FUNCTION_BLOCK FB111
TITLE =Get Velocity Must
//*****************************************************************************
//* maxon motor ag
//* R&D
//* all rights reserved
//*****************************************************************************
//* Summary:  Read demand value of velocity
//*
//* Remarks:
//*
//* Created under: STEP7 REV5.2+SP1
//*****************************************************************************
//* History:
//* 19.05.2004 | INA   first release
//*
//*
//*****************************************************************************
//

AUTHOR:INA
FAMILY:Velocity
NAME:SetVeloM
VERSION:00.01


VAR_INPUT

Read : BOOL //A rising edge start the command

  NodeID : BYTE //Adress of the maxon device

END_VAR
VAR_OUTPUT
  Done : BOOL //Data valid flag is TRUE if data were available

  Err : BOOL //Error flag is TRUE if an Error has occured, see ErrNo for more details

  ErrNo : DINT //Contains detailed error information

  VelocityMust : DINT //Velocity demand value

END_VAR
VAR
  xEdgeMerker : BOOL //Edge Merker

  xEdgeFlag : BOOL //Edge Flag

  xStep : INT
END_VAR

BEGIN

NETWORK
TITLE = Activate the service function
//

// SDO Read "Get Velocity Must"

       U    #Read
       FP   #xEdgeFlag                   // recognize a positiv edge of the Read signal
       =    #xEdgeMerker                 // and set the xEdgeMerker for one cycle to true

       L    #xStep
       L    0
       ==I
       U    #xEdgeMerker
       SPB  nstp                         // iStep = 1 -> fnc1

       L    #xStep                       // jump list
       SPL  List
       SPA  rdef
       SPA  fnc1
       SPA  fncE
List  :SPA  rdef

rdef  :NOP  0
       R    #Done                        // reset Done
       R    #Err                         // reset Error
       L    0
       T    #xStep                       // iStep = 0
       SPA  end

fnc1  :NOP  0
       CALL FC1
         NodeID:=#NodeID
         Index:=DW#16#0000206B
         SubIndex:=DW#16#00000000
         RET_VAL:=#Done
         Err:=#Err
         ErrNo:=#ErrNo

       L    DB219.DBD10
       T    #VelocityMust

fncE  :NOP  0
       L    0
       T    #xStep
       SPA  end

nstp  :NOP  0
       L    #xStep
       INC            1
       T    #xStep

end   :NOP  0
END_FUNCTION_BLOCK
